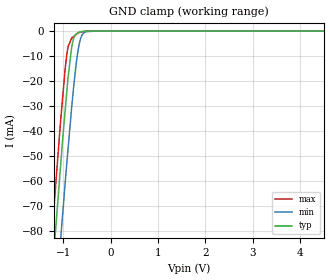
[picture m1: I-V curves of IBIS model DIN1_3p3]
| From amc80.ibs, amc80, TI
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|NOTES   Model TERM split into two Models TERM_3p3 and TERM_5
|   to accomodate vast voltage range of 3.0V - 5.5V
|   TERM_3p3 operates in voltage range of 3 - 3.3 - 3.6
|   TERM_5 operates in voltage range of 4.5 - 5 - 5.5
|   DIN1 model
[Model]  DIN1_3p3
Model_type   Input
Vinl = 0.8
Vinh = 2.0
|   typ   min   max
|   (nom PVT)   (Fast PVT)   (slow PVT)
C_comp   5.573E-13   5.347E-13   6.082E-13
| Where   nom PVT is  Nominal Process, 3.3V, 27C
|   Fast PVT is Strong Process, 3.6V, -40C
|   Slow PVT is Weak Process, 3.0V, 125C
|C_comp - from L-C Tank method, L = 1nH, peak frequency
[Voltage Range]   3.3   3   3.6
[Temperature Range]   27   125   -40
[Power Clamp Reference]   3.3   3   3.6
[GND Clamp Reference]   0   0   0
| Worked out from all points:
|   GND clamp passes 1 mA (typ) near -0.72 V on its own axis
[GND Clamp]
|   Voltage   I(typ)   I(min)   I(max)
-3.3V     -646.6mA   -664.3mA   -639.2mA
-1.233V   -97.24mA   -127mA     -79.71mA
-1.171V   -81.49mA   -111.4mA   -64.21mA
-1.064V   -55.52mA   -85.13mA   -37.57mA
-1.014V   -43.36mA   -73.27mA   -26.64mA
-924.4mV  -23.98mA   -52.53mA   -9.169mA
-806.3mV  -4.749mA   -27.19mA   -2.534mA
-736.8mV  -1.299mA   -14.5mA    -1.496mA
-675.7mV  -477.6uA   -6.375mA   -602.2uA
-578.1mV  -79.56uA   -895.2uA   -247.7uA
-330.4mV  -11.18uA   -1.944uA   -11.32uA
6.59V     0A         0A         0A
[POWER Clamp]
|   SCR cell for ESD function. Effects occurr above VDD x 2
|   Voltage   I(typ)   I(min)   I(max)
-3.3V     0A         0A         0A
0V        0A         0A         0A
6.6V      0A         0A         0A
